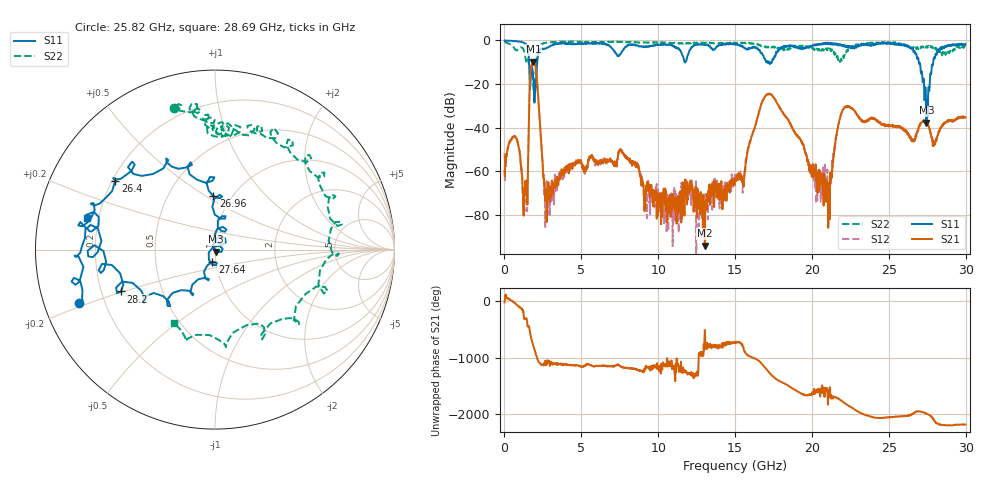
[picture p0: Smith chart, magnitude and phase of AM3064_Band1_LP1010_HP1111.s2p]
# Hz S DB R 50.0
!freq dBS11 angS11 dBS21 angS21 dBS12 angS12 dBS22 angS22
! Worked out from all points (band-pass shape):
!   1600 points, 10 MHz to 29.98 GHz, reference 50 ohm
!   highest |S21| = -9.67 dB at 1.884 GHz (marker M1); lowest = -93.9 dB at 13.04 GHz (marker M2)
!   |S21| within 3 dB of the highest: 1.722 GHz to 2.04 GHz (317.3 MHz wide, 16.9 % of centre)
!   lowest |S11| = -37.7 dB at 27.45 GHz (marker M3), VSWR 1.03, Z = 50.7 - j1.13 ohm
!   |S11| at or under -10 dB: 1.6 GHz to 2.13 GHz (529.9 MHz wide, 28.4 % of centre); 17.22 GHz to 17.39 GHz (166.5 MHz wide, 0.962 % of centre); 26.95 GHz to 27.89 GHz (939.1 MHz wide, 3.42 % of centre)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
!   |S22| runs from -24.6 to -0.4 dB; largest |S21 - S12| = 0.0057
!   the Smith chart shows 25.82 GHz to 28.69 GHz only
!   S11 on the Smith chart (normalised r, x): 25.82 GHz: 0.11, -0.19; 26.4 GHz: 0.21, +0.30; 26.96 GHz: 0.82, +0.54; 27.64 GHz: 0.96, -0.13; 28.2 GHz: 0.28, -0.20; 28.69 GHz: 0.15, +0.12
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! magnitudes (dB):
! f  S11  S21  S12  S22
! 10 MHz  0.0  -59.7  -51.5  -0.4
! 722.3 MHz  -0.3  -44.4  -44.4  -4.4
! 1.36 GHz  -1.5  -65.1  -65.8  -7.9
! 1.884 GHz  -17.8  -9.7  -9.7  -21.3
! 2.803 GHz  -3.2  -71.1  -76.0  -1.0
! 5.015 GHz  -1.4  -56.3  -56.7  -0.8
! 10 GHz  -2.0  -69.9  -68.4  -0.9
! 13.04 GHz  -2.0  -93.9  -78.5  -1.2
! 15 GHz  -1.8  -64.7  -63.4  -1.5
! 17.18 GHz  -9.8  -24.4  -24.3  -3.1
! 19.99 GHz  -2.7  -61.9  -62.5  -3.3
! 21.08 GHz  -1.8  -78.5  -67.4  -4.1
! 22.2 GHz  -2.3  -30.3  -30.4  -6.3
! 25 GHz  -1.0  -39.4  -39.2  -1.0
! 25.82 GHz  -1.8  -40.4  -40.4  -1.7
! 26.4 GHz  -3.4  -44.3  -43.9  -3.1
! 26.96 GHz  -10.5  -39.2  -39.9  -3.1
! 27.45 GHz  -37.7  -38.0  -37.4  -2.5
! 27.64 GHz  -23.1  -40.3  -40.5  -3.3
! 28.2 GHz  -4.8  -43.3  -43.1  -4.4
! 28.69 GHz  -2.7  -37.6  -37.4  -6.6
! 29.98 GHz  -1.7  -35.2  -35.4  -3.1
